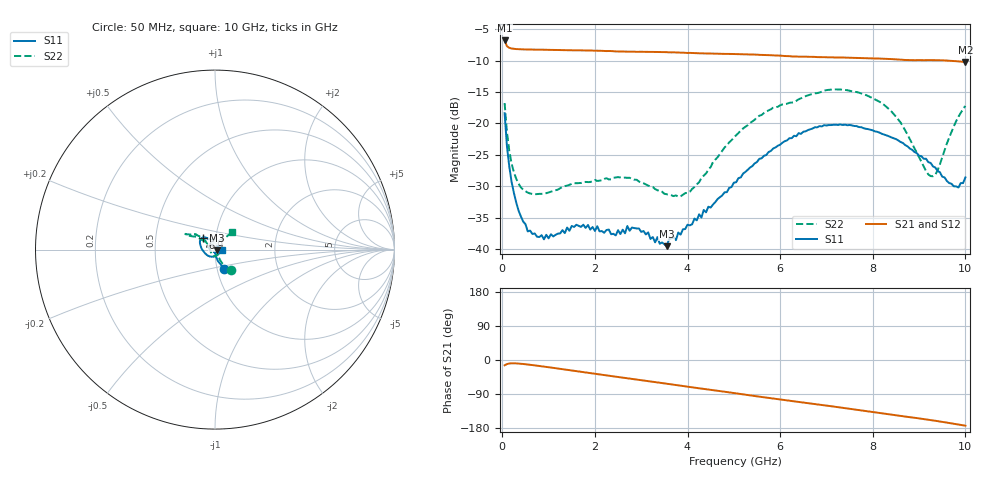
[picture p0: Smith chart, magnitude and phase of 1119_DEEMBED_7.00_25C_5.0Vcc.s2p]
!Hittite Microwave Corp.
!Digital Attenuator/PhaseShifter Rev 1.4.0
!Filename: C:\DATA\DATA\1119_DEEMBED_7.00_25C_5.0Vcc.s2p
!VNA ID: Agilent Technologies,N5224A,MY51441122,A.10.45.03
!Device type:
!2 Port Calibration.
!Temp(C): 25
!Lot Number:
!Serial Number:
!Operator:
!Misc:
!Attenuator:  7.000
# GHZ S DB R 50.0
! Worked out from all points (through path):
!   200 points, 50 MHz to 10 GHz, reference 50 ohm
!   highest |S21| = -6.79 dB at 50 MHz (marker M1); lowest = -10.2 dB at 10 GHz (marker M2)
!   group delay of S21, straight-line fit = 46.7 ps
!   lowest |S11| = -39.5 dB at 3.55 GHz (marker M3), VSWR 1.02, Z = 51 - j0.36 ohm
!   |S11| at or under -10 dB: start of sweep to end of sweep
!   |S22| runs from -31.6 to -14.6 dB; largest |S21 - S12| = 0.0013
!   S11 on the Smith chart (normalised r, x): 50 MHz: 1.08, -0.24; 6.9 GHz: 0.87, +0.12; 10 GHz: 1.08, -0.00
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0.05  -18.37 -64.2  -6.79 -14.0  -6.79 -14.0  -16.76 -52.8
0.1  -23.58 -75.5  -7.70 -10.8  -7.70 -10.8  -21.34 -62.3
0.2  -29.28 -82.3  -8.07 -8.7  -8.07 -8.7  -26.35 -64.0
0.35  -33.85 -84.3  -8.18 -9.4  -8.18 -9.4  -29.57 -60.0
0.55  -37.19 -88.7  -8.23 -11.9  -8.23 -11.9  -31.02 -58.2
0.9  -38.45 -94.4  -8.27 -17.4  -8.27 -17.4  -31.17 -61.8
1.75  -36.12 -103.3  -8.37 -31.9  -8.38 -31.9  -29.34 -78.9
2.45  -37.83 -84.0  -8.53 -44.0  -8.53 -44.1  -28.61 -97.5
2.7  -36.33 -73.2  -8.57 -48.1  -8.58 -48.2  -28.66 -105.2
2.95  -36.72 -72.6  -8.59 -52.2  -8.60 -52.2  -29.25 -115.9
3.4  -39.15 -44.8  -8.63 -60.0  -8.64 -60.0  -30.68 -133.3
3.55  -39.54 -19.5  -8.65 -62.7  -8.66 -62.8  -31.28 -139.8
4.05  -36.23 12.7  -8.77 -71.2  -8.78 -71.2  -30.87 -179.7
5.05  -29.36 82.3  -8.96 -88.0  -8.98 -88.0  -21.87 136.9
5.85  -23.99 116.9  -9.16 -101.9  -9.18 -102.0  -17.49 141.4
6.7  -20.81 132.8  -9.40 -115.5  -9.42 -115.5  -15.30 149.9
6.9  -20.48 135.9  -9.45 -118.7  -9.46 -118.7  -14.93 151.9
7.65  -20.42 152.3  -9.57 -131.3  -9.58 -131.4  -15.00 153.1
8.35  -22.05 169.8  -9.74 -143.5  -9.75 -143.5  -17.72 146.7
9.3  -26.84 -122.1  -9.92 -159.4  -9.94 -159.4  -28.41 104.1
9.75  -30.01 -49.2  -10.07 -168.2  -10.08 -168.3  -20.45 48.3
10  -28.60 -0.5  -10.22 -173.3  -10.23 -173.3  -17.21 45.5
